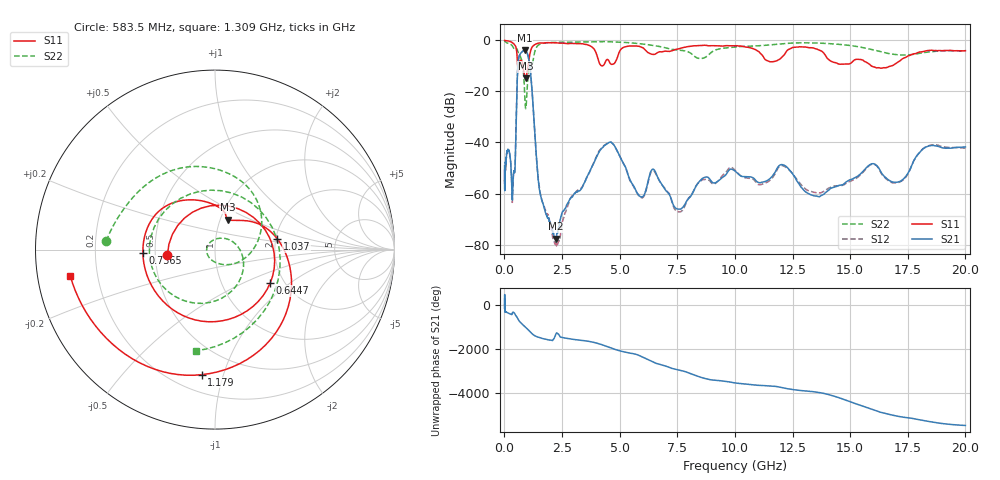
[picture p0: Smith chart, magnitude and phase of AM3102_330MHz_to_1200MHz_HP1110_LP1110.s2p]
! Date/Time: Tue, Sep 11, 2018 5:23 PM
! Network Analyzer: Agilent Technologies E8362B Rev: A.07.50.63
! Sweep from 0.010 to 20.000 GHz, 1601 Points, Sweep Type: LOG
! Power Supply: 4.949 V, 0.001 A
# Hz S DB R 50
!freq MagS11 AngS11 MagS21 AngS21 MagS12 AngS12 MagS22 AngS22
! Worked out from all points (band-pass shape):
!   1601 points, 10 MHz to 20 GHz, reference 50 ohm
!   highest |S21| = -3.83 dB at 873.8 MHz (marker M1); lowest = -77.7 dB at 2.228 GHz (marker M2)
!   |S21| within 3 dB of the highest: 620.3 MHz to 1.047 GHz (426.7 MHz wide, 51.2 % of centre)
!   lowest |S11| = -14.8 dB at 925.1 MHz (marker M3), VSWR 1.44, Z = 54.4 + j18.7 ohm
!   |S11| at or under -10 dB: 573.3 MHz to 628.3 MHz (55.03 MHz wide, 9.16 % of centre); 803.6 MHz to 1.021 GHz (217.2 MHz wide, 23.8 % of centre); 15.92 GHz to 16.8 GHz (883.2 MHz wide, 5.4 % of centre)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
!   |S22| runs from -26.7 to -0.2 dB; largest |S21 - S12| = 0.0082
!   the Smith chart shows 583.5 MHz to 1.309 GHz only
!   S11 on the Smith chart (normalised r, x): 583.5 MHz: 0.58, -0.04; 644.7 MHz: 1.70, -0.72; 736.5 MHz: 0.43, -0.02; 1.037 GHz: 2.04, +0.28; 1.179 GHz: 0.31, -0.85; 1.309 GHz: 0.10, -0.09
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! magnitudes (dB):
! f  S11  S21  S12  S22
! 10 MHz  -0.1  -49.1  -50.8  -0.2
! 35.55 MHz  -0.1  -51.8  -52.5  -0.5
! 126.4 MHz  -0.2  -43.3  -43.3  -1.0
! 257.7 MHz  -0.5  -46.5  -46.2  -1.5
! 342.8 MHz  -1.0  -62.4  -63.2  -2.2
! 447.2 MHz  -1.8  -51.8  -51.3  -3.6
! 583.5 MHz  -11.5  -10.2  -10.2  -4.3
! 644.7 MHz  -8.9  -6.0  -6.2  -5.6
! 736.5 MHz  -7.9  -4.8  -4.8  -7.3
! 873.8 MHz  -13.5  -3.8  -3.9  -19.5
! 925.1 MHz  -14.8  -4.0  -4.1  -26.7
! 1.037 GHz  -9.1  -6.4  -6.4  -12.6
! 1.179 GHz  -3.1  -17.2  -17.1  -9.6
! 1.309 GHz  -1.7  -34.6  -35.0  -4.8
! 1.59 GHz  -1.0  -61.4  -61.2  -1.3
! 2.228 GHz  -0.9  -77.7  -79.4  -0.8
! 4.436 GHz  -7.6  -40.6  -40.5  -0.5
! 5.652 GHz  -2.2  -57.8  -58.1  -1.1
! 7.588 GHz  -3.3  -66.1  -67.2  -3.9
! 12.09 GHz  -6.1  -48.8  -49.1  -1.3
! 13.55 GHz  -3.4  -61.0  -59.7  -1.1
! 20 GHz  -4.0  -41.7  -42.3  -4.2
